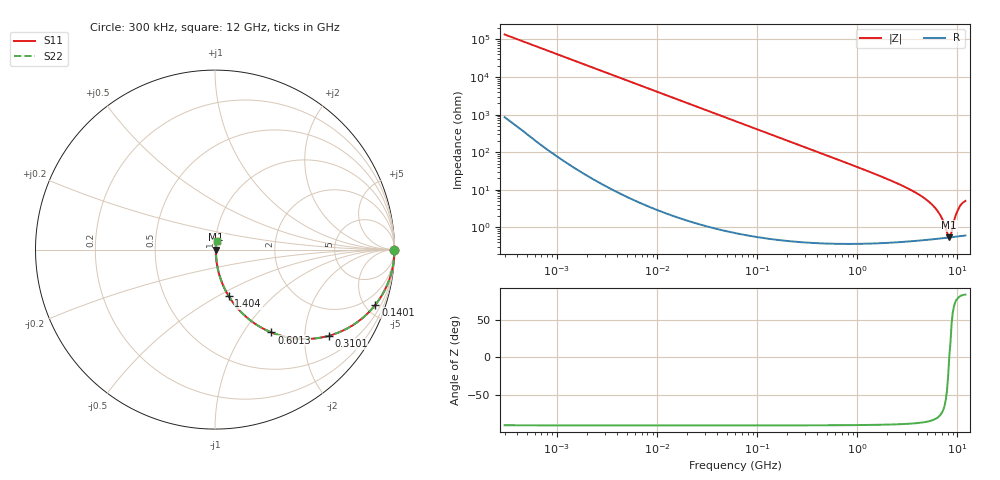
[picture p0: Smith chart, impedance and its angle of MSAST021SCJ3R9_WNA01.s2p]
! MSAST021SCJ3R9_WNA01  S-PARAMETER MODEL  ( General Type )
! Model Generated by TAIYO YUDEN Corporation (http://www.ty-top.com)
! Version 2.0
! TAIYO YUDEN Control No. 181101
! Copyright(c) 2015 TAIYO YUDEN CO.,LTD. All Rights Reserved.
! Product Description (link to TY-COMPAS)
! https://ds.yuden.co.jp/TYCOMPAS/or/detail?pn=MSAST021SCJ3R9BWNA01&u=M
! Products Name : Multilayer Ceramic Capacitors
! Characteristics :
!  Capacitance : 3.9 pF , Rated Voltage : 25V , TCC : CJ / C0J
!  Case Size : 0.25 x 0.125 / 0.0098 x 0.0049 [mm/inch] , Thickness : 0.125 / 0.0049 [mm/inch]
!  (Conditions: Temperature = 25 degC , DC Bias Current/Voltage = 0A / 0V)
! External Node Assignments :
!  1  o---| |---o  2
! GND o---------o GND
! Frequency Range : 0.3MHz  -  12000MHz  [ 401 STEP ]
# MHz S RI R 50
! Freq[MHz].  S11 Real  S11 Imag  S21 Real  S21 Imag  S12 Real  S12 Imag  S22 Real  S22 Imag
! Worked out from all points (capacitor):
!   401 points, 300 kHz to 12 GHz, reference 50 ohm
!   read as one part in series: C = 3.9 pF near 316.3 kHz
!   lowest |Z| = 537 mohm at 8.282 GHz (marker M1)
!   series resonance near 8.278 GHz, so ESL is about 95 pH
!   S11 on the Smith chart (normalised r, x): 300 kHz: open; 140.1 MHz: 1.01, -5.83; 310.1 MHz: 1.01, -2.63; 601.3 MHz: 1.01, -1.35; 1.404 GHz: 1.01, -0.56; 12 GHz: 1.01, +0.10
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0.3  1 -0.000735  5.17e-06 0.000735  5.17e-06 0.000735  1 -0.000735
1.769972  1 -0.00434  2.42e-05 0.00434  2.42e-05 0.00434  1 -0.00434
10.44266  0.9993 -0.0256  0.000672 0.0256  0.000672 0.0256  0.9993 -0.0256
60  0.9787 -0.1439  0.0213 0.1439  0.0213 0.1439  0.9787 -0.1439
140.0606  0.8942 -0.3068  0.1058 0.3068  0.1058 0.3068  0.8942 -0.3068
310.0777  0.6329 -0.4805  0.3671 0.4805  0.3671 0.4805  0.6329 -0.4805
353.9943  0.5695 -0.4935  0.4305 0.4935  0.4305 0.4935  0.5695 -0.4935
601.3112  0.314 -0.4614  0.686 0.4614  0.686 0.4614  0.314 -0.4614
918.7169  0.1635 -0.3657  0.8365 0.3657  0.8365 0.3657  0.1635 -0.3657
1403.667  0.0768 -0.2597  0.9232 0.2597  0.9232 0.2597  0.0768 -0.2597
2088.533  0.0359 -0.1757  0.9641 0.1757  0.9641 0.1757  0.0359 -0.1757
3740.715  0.0117 -0.0854  0.9883 0.0854  0.9883 0.0854  0.0117 -0.0854
5420.343  0.00654 -0.0425  0.9935 0.0425  0.9935 0.0425  0.00654 -0.0425
6699.894  0.00545 -0.0208  0.9946 0.0208  0.9946 0.0208  0.00545 -0.0208
7254.098  0.0053 -0.0129  0.9947 0.0129  0.9947 0.0129  0.0053 -0.0129
7854.144  0.00528 -0.00512  0.9947 0.00512  0.9947 0.00512  0.00528 -0.00512
8281.503  0.00534 4.58e-05  0.9947 -4.58e-05  0.9947 -4.58e-05  0.00534 4.58e-05
8732.115  0.00546 0.00525  0.9945 -0.00525  0.9945 -0.00525  0.00546 0.00525
9454.42  0.00587 0.0173  0.9941 -0.0173  0.9941 -0.0173  0.00587 0.0173
10236.47  0.00662 0.03  0.9934 -0.03  0.9934 -0.03  0.00662 0.03
11083.22  0.00764 0.042  0.9924 -0.042  0.9924 -0.042  0.00764 0.042
12000  0.00848 0.0494  0.9915 -0.0494  0.9915 -0.0494  0.00848 0.0494
